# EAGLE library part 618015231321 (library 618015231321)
Wurth Elektronik 618 Series 2.77 mm, 2.84 mm Pitch 15 Way Right Angle Through Hole Mount PCB D-sub Connector, Socket Source: Datasheet
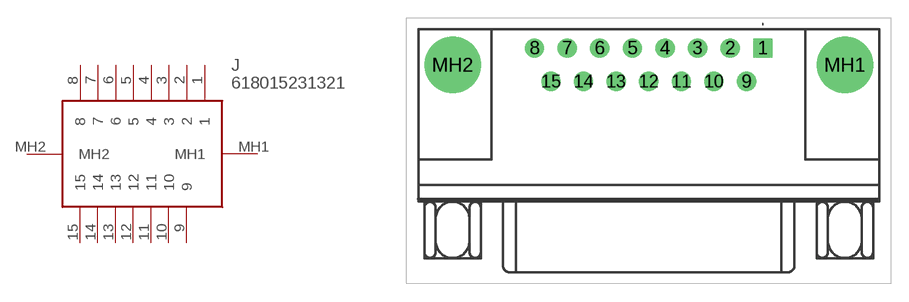
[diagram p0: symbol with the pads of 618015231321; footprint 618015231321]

Designator prefix J

## 618015231321 (Description: Wurth Elektronik 618 Series 2.77 mm, 2.84 mm Pitch 15 Way Right Angle Through Hole Mount PCB D-sub Connector, Socket; Height: 12.85mm; Manufacturer_Name: Wurth Elektronik; Manufacturer_Part_Number: 618015231321; Mouser_Part_Number: 710-618015231321; Mouser_Price-Stock: https://www.mouser.co.uk/ProductDetail/Wurth-Elektronik/618015231321?qs=ZtY9WdtwX559EG5kq7agHA%3D%3D)  [618015231321]
1  1
2  2
3  3
4  4
5  5
6  6
7  7
8  8
9  9
10  10
11  11
12  12
13  13
14  14
15  15
MH1  MH1
MH2  MH2

## Footprint 618015231321 (pad centres in mm)
618015231321-2
drill 1.09 pad 1.635 square: 1 0,0
drill 1.09 pad 1.635: 2 -2.77,0; 3 -5.54,0; 4 -8.31,0; 5 -11.08,0; 6 -13.85,0; 7 -16.62,0; 8 -19.39,0; 9 -1.385,-2.84; 10 -4.155,-2.84; 11 -6.925,-2.84; 12 -9.695,-2.84; 13 -12.465,-2.84; 14 -15.235,-2.84; 15 -18.005,-2.84
drill 3.2 pad 4.8: MH1 6.965,-1.42; MH2 -26.355,-1.42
